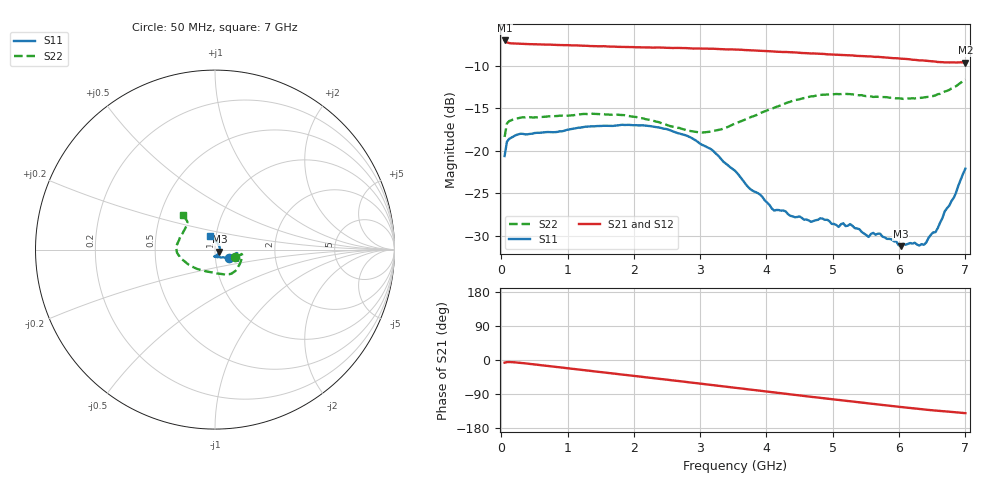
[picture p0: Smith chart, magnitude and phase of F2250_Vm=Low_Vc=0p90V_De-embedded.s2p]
! Integrated Device Technology
! Corporate Headquarters
! 6024 Silver Creek Valley Road
! San Jose, CA 95138  USA
! Phone:  1-408-284-8200
! Toll Free:  1-800-223-1366
! Webpage:  http://www.idt.com/
! Timing and RF Division
! 515 Groton Road, Suite 102
! Westford, MA 01886-6024
! Device:  F2250
! Description: Voltage Variable RF Attenuator
! Frequency:  50.0 -  6000.00 MHz
! Package:  3x3 mm Thin QFN Plastic Package: 16 pin
! Ports:  2 RF, 3 DC
!  Pin  1  = GND
!  Pin  2  = NC
!  Pin  3  = RF1  = Port 1
!  Pin  4  = NC
!  Pin  5  = GND
!  Pin  6  = GND
!  Pin  7  = GND
!  Pin  8  = GND
!  Pin  9  = NC
!  Pin 10  = RF2  = Port 2
!  Pin 11  = NC
!  Pin 12  = GND
!  Pin 13  = GND
!  Pin 14  = VCNTRL
!  Pin 15  = VDD
!  Pin 16  = VMODE
! Vcntrl:  0.900 Volts
! Vmode:  +0.000 Volts
! Vdd:  +3.30  Volts
! Current:  1.176 mA
! Data:  The device was measured on a the F2250 evaluation board which has
!  individual transmission lines to the RF pins.  Data was collected
!  using a calibrated network analyzer.  The evaluation board was
!  de-embedded using a TRL calibration technique.
!  The reference plane is the edge of the package pin.
! Misc:  SN 10
!  Action Tracker AT0258
! Date Measured:  2014-11-26
! Date:  2015-10-15  MJV
! Note:
!  Integrated Device Technology supplies this data as a sample of measured
!  data at the package pin for this product.  Your particular data for this
!  product may vary.
!  Data was taken at 25 degrees C.
!  Integrated Device Technology reserves the right to change this data at anytime.
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# GHz S dB R 50
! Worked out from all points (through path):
!   201 points, 50 MHz to 7 GHz, reference 50 ohm
!   highest |S21| = -7.05 dB at 50 MHz (marker M1); lowest = -9.6 dB at 7 GHz (marker M2)
!   group delay of S21, straight-line fit = 56.1 ps
!   lowest |S11| = -31.2 dB at 6.027 GHz (marker M3), VSWR 1.06, Z = 52.5 - j1.27 ohm
!   |S11| at or under -10 dB: start of sweep to end of sweep
!   |S22| runs from -18.4 to -11.6 dB; largest |S21 - S12| = 0.0011
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0.05  -20.63 -29.8  -7.05 -7.0  -7.04 -7.0  -18.39 -20.6
0.08475  -18.96 -14.9  -7.29 -5.5  -7.29 -5.5  -16.80 -11.5
0.22375  -18.16 -9.0  -7.41 -6.5  -7.42 -6.5  -16.25 -11.2
1.2315  -17.23 -23.4  -7.67 -26.5  -7.68 -26.5  -15.69 -42.3
1.857  -16.98 -25.9  -7.80 -39.0  -7.81 -39.0  -15.83 -56.7
2.37825  -17.27 -25.6  -7.88 -49.5  -7.89 -49.5  -16.66 -70.2
3.0385  -19.35 -27.8  -8.00 -63.1  -7.99 -63.1  -17.86 -101.5
3.525  -22.35 -37.4  -8.12 -73.4  -8.12 -73.4  -16.83 -130.4
4.11575  -27.03 -66.5  -8.35 -85.7  -8.34 -85.7  -14.96 -157.1
4.7065  -28.26 -93.2  -8.58 -97.8  -8.57 -97.8  -13.61 -173.5
4.8455  -27.98 -92.9  -8.63 -100.6  -8.63 -100.6  -13.44 -176.4
5.08875  -28.96 -90.7  -8.75 -105.5  -8.74 -105.5  -13.36 177.8
5.2625  -28.63 -84.1  -8.80 -109.0  -8.80 -109.0  -13.36 173.9
5.5405  -30.14 -69.5  -8.92 -114.5  -8.91 -114.6  -13.57 167.0
5.61  -29.66 -63.8  -8.95 -115.9  -8.96 -115.9  -13.69 165.3
5.85325  -30.36 -43.9  -9.09 -120.6  -9.09 -120.7  -13.77 158.8
6.027  -31.22 -26.1  -9.19 -124.0  -9.18 -124.1  -13.87 153.5
6.3745  -31.06 27.2  -9.41 -130.6  -9.43 -130.6  -13.75 141.9
6.54825  -29.57 57.6  -9.53 -133.4  -9.54 -133.4  -13.50 137.2
6.68725  -27.15 76.2  -9.63 -135.4  -9.63 -135.5  -13.05 134.3
6.82625  -25.53 93.8  -9.62 -137.6  -9.63 -137.6  -12.56 133.9
7  -22.11 111.4  -9.65 -140.2  -9.65 -140.3  -11.64 133.3
